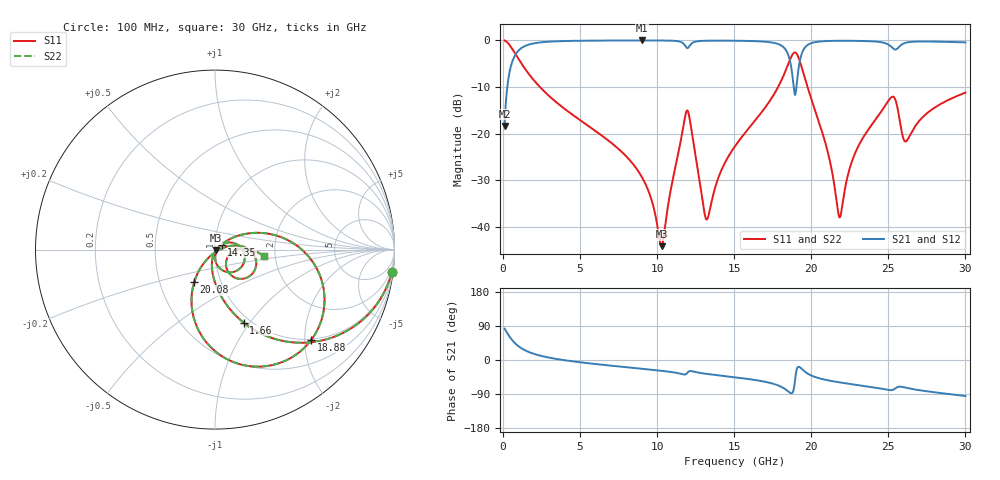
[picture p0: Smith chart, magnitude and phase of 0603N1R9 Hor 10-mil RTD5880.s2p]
# GHz S MA R 50
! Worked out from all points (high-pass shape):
!   3201 points, 100 MHz to 30 GHz, reference 50 ohm
!   highest |S21| = -0.04 dB at 9.023 GHz (marker M1); lowest = -18.3 dB at 100 MHz (marker M2)
!   |S21| within 3 dB of the highest: 812.6 MHz to 18.5 GHz (17.68 GHz wide, 183 % of centre); 19.36 GHz to end of sweep
!   lowest |S11| = -44.1 dB at 10.28 GHz (marker M3), VSWR 1.01, Z = 50.5 - j0.342 ohm
!   |S11| at or under -10 dB: 2.386 GHz to 17.85 GHz (15.46 GHz wide, 153 % of centre); 19.76 GHz to end of sweep
!   |S22| runs from -44.1 to -0.1 dB; largest |S21 - S12| = 0
!   S11 on the Smith chart (normalised r, x): 100 MHz: 1, -16; 1.66 GHz: 0.93, -0.93; 14.35 GHz: 1.08, +0.06; 18.88 GHz: 0.99, -2.16; 20.08 GHz: 0.75, -0.28; 30 GHz: 1.74, -0.14
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0.1  0.9926 -7.2  0.121 82.8  0.121 82.8  0.9926 -7.2
0.6045625  0.8043 -38.1  0.5937 51.8  0.5937 51.8  0.8043 -38.1
1.660406  0.4376 -68.5  0.8978 21.3  0.8978 21.3  0.4376 -68.5
5.089563  0.1361 -95.3  0.9879 -6.4  0.9879 -6.4  0.1361 -95.3
9.023281  0.03395 -105.9  0.995 -23.2  0.995 -23.2  0.03395 -105.9
10.06978  0.009032 -78.9  0.9942 -27.6  0.9942 -27.6  0.009032 -78.9
10.28469  0.006236 -32.9  0.9936 -28.6  0.9936 -28.6  0.006236 -32.9
11.9105  0.1745 -18.8  0.8318 -36.0  0.8318 -36.0  0.1745 -18.8
13.18125  0.01212 -34.1  0.9877 -36.5  0.9877 -36.5  0.01212 -34.1
14.34922  0.04706 37.0  0.99 -42.2  0.99 -42.2  0.04706 37.0
15.05  0.0733 37.3  0.9881 -45.6  0.9881 -45.6  0.0733 37.3
18.07737  0.3772 10.5  0.8735 -71.3  0.8735 -71.3  0.3772 10.5
18.88094  0.7351 -43.0  0.2933 -73.1  0.2933 -73.1  0.7351 -43.0
19.39484  0.5033 -97.0  0.7288 -24.0  0.7288 -24.0  0.5033 -97.0
20.03956  0.2253 -121.8  0.9364 -41.6  0.9364 -41.6  0.2253 -121.8
20.07694  0.2157 -122.5  0.9404 -42.3  0.9404 -42.3  0.2157 -122.5
21.84291  0.01267 -56.6  0.987 -59.1  0.987 -59.1  0.01267 -56.6
22.87072  0.06335 13.6  0.9854 -65.2  0.9854 -65.2  0.06335 13.6
25.01978  0.2267 -10.4  0.8951 -79.2  0.8951 -79.2  0.2267 -10.4
25.44025  0.2339 -42.7  0.7947 -75.3  0.7947 -75.3  0.2339 -42.7
26.14103  0.08251 -26.5  0.9413 -73.2  0.9413 -73.2  0.08251 -26.5
30  0.2753 -7.5  0.9492 -95.1  0.9492 -95.1  0.2753 -7.5
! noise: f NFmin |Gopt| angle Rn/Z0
0.1  0.0004506  0.9489  0.9614  0.001978
3.417  0.004032  0.8099  9.874  0.004387
6.743  0.006892  0.7845  19  0.006395
10.06  0.01108  0.7997  27.99  0.0108
13.39  0.01758  0.8309  36.98  0.01973
16.7  0.02273  0.838  45.64  0.02526
20.03  0.04148  0.8918  54.52  0.06604
23.35  0.02573  0.8082  62.73  0.02044
26.67  0.03932  0.8548  70.99  0.03845
30  0.02741  0.7785  78.57  0.01534
